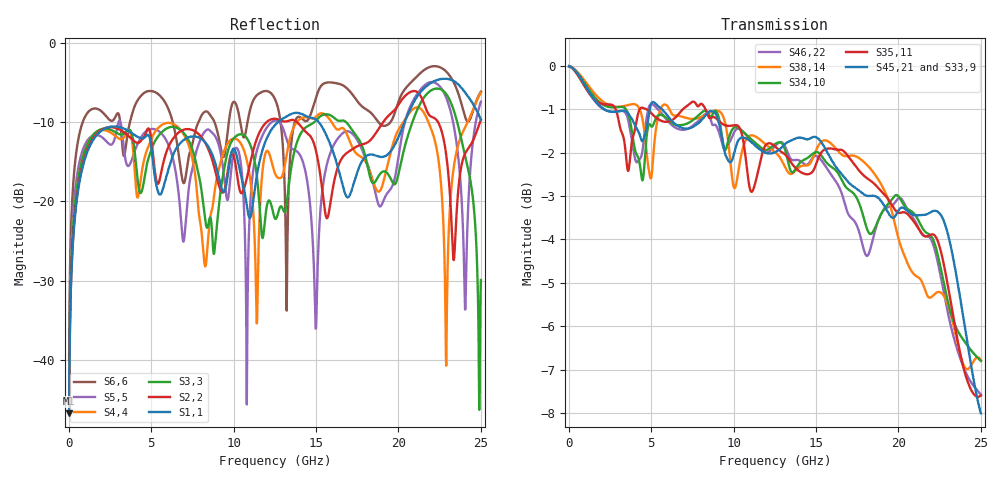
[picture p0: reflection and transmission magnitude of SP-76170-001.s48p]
! IMPORTANT NOTE: This model should not be used to evaluate
! electrical signals with a greater than 25 GHz. of frequency content.
! Please apply appropriate analysis techniques when reviewing the results of
! your simulations.
!  COPYRIGHT 2008, BY MOLEX INCORPORATED
!  ALL INTERNATIONAL RIGHTS RESERVED
!  THIS FILE CONTAINS MOLEX INCORPORATED CONFIDENTIAL INFORMATION
! >>>>>>>>>>>>>>>>  USER AGREEMENT  <<<<<<<<<<<<<<<<<<<
! The information on this media is the property of MOLEX Incorporated
! and  has been provided to you free of charge. Molex does not
! guarantee that the information is error-free, nor does MOLEX  make
! any representations, warranty or guarantee that the information is
! accurate, correct, reliable or up-to-date. MOLEX expressly
! disclaims all implied warranties regarding this information,
! including but not limited to any implied  warranties of
! merchantability or fitness for a particular purpose. MOLEX does
! not warrant that the media will work correctly in your multi- user
! or network environment.
! MOLEX will in no case be liable for your use, or the results of
! your use, of the software and other information contained on this
! media or  any accompanying written materials.  IT IS YOUR
! RESPONSIBILITY TO VERIFY THE RESULTS OF YOUR USE OF THIS
! INFORMATION IN YOUR OWN PARTICULAR ENGINEERING AND PRODUCT
! ENVIRONMENT, AND YOU ASSUME THE ENTIRE RISK OF DOING SO OR
! FAILING TO DO SO.  In no event will MOLEX be liable for any
! direct, indirect, incidental or consequential damages arising from
! your use of, or your inability to use, software, product simulations
! and other information contained on this media or any accompanying
! written materials.
! This model has not been validated with empirical data.
! This model was solved using HFSS.  TDR results can run 5-8 ohms low
! Touchstone file from project 3PAIRS_4WAFER_RAF_RAM_100_Ohm_PM
! Exported from HFSS 13.0.0
! Variables:
!  wp_DC_xsize = 0.8168mm
!  wp_DC_ysize = 0.6398mm
!  wplen = 1mm
!  wpvac_BP_xsize = 0.6366mm
!  wpvac_BP_ysize = 0.4866mm
! Terminal data exported
! Port[1] = B1_T1
! Port[2] = C1_T1
! Port[3] = E1_T1
! Port[4] = F1_T1
! Port[5] = H1_T1
! Port[6] = J1_T1
! Port[7] = A2_T1
! Port[8] = B2_T1
! Port[9] = D2_T1
! Port[10] = E2_T1
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# GHZ S MA R 50.000000
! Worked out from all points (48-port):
!   1250 points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, 20 MHz to 25 GHz, reference 50 ohm
!   strongest paths, dB at 20 MHz, 6.26 GHz, 12.52 GHz, 18.76 GHz, 25 GHz:
!     S45,21: 0.0, -1.3, -2.0, -3.0, -8.0
!     S33,9: 0.0, -1.1, -1.9, -3.1, -7.3
!     S35,11: 0.0, -1.3, -1.9, -2.8, -7.6
!     S34,10: 0.0, -1.3, -1.8, -3.6, -6.8
!     S38,14: 0.0, -1.1, -2.0, -2.6, -6.8
!     S46,22: 0.0, -1.4, -1.8, -3.6, -7.6
!   lowest |S11| = -46.7 dB at 20 MHz (marker M1), VSWR 1.01, Z = 50.1 + j0.457 ohm
!   |S11| at or under -10 dB: start of sweep to 12.7 GHz; 15.16 GHz to 20.37 GHz (5.212 GHz wide, 29.3 % of centre)
